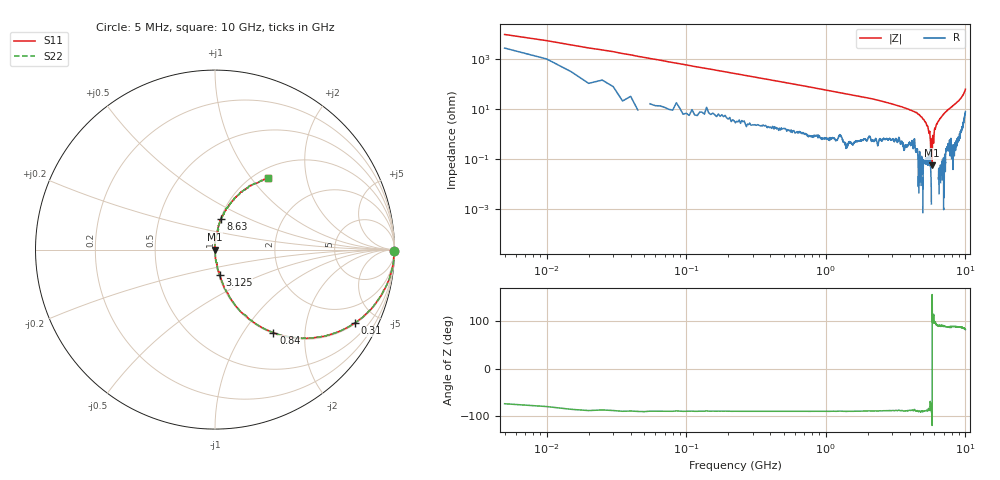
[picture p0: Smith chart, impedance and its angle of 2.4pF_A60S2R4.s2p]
! Amotech Co.,Ltd.
! http://www.amotech.co.kr/
! Part Number: A60S2R4
! These Parameters are Measured in Series Mode Connection
! Operation Temp=25[degC], DC Bias Voltage=0[V]
! Freq. Start=5[MHz] Stop=10[GHz], 2000[Steps]
! Date: Monday, July 13, 2020, 01:52:19
# GHZ S RI R 50.000000
!Freq.(Hz) S11(Real) S11(Imag) S21(Real) S21(Imag) S12(Real) S12(Imag) S22(Real) S22(Imag)
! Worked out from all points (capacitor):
!   2000 points, 5 MHz to 10 GHz, reference 50 ohm
!   read as one part in series: C = 2.74 pF near 55 MHz
!   lowest |Z| = 54.2 mohm at 5.785 GHz (marker M1)
!   series resonance near 5.784 GHz, so ESL is about 280 pH
!   S11 on the Smith chart (normalised r, x): 5 MHz: open; 310 MHz: 1.05, -3.78; 840 MHz: 1.02, -1.38; 3.125 GHz: 1.01, -0.29; 8.63 GHz: 1.01, +0.35; 10 GHz: 1.16, +1.22
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0.005  0.997 -0.00986  0.00304 0.00986  0.00304 0.00986  0.997 -0.00986
0.065  0.9863 -0.1091  0.0137 0.1091  0.0137 0.1091  0.9863 -0.1091
0.105  0.9668 -0.1742  0.0332 0.1742  0.0332 0.1742  0.9668 -0.1742
0.31  0.7781 -0.4094  0.2219 0.4094  0.2219 0.4094  0.7781 -0.4094
0.84  0.325 -0.4621  0.675 0.4621  0.675 0.4621  0.325 -0.4621
1.675  0.1039 -0.2975  0.8961 0.2975  0.8961 0.2975  0.1039 -0.2975
3.125  0.0262 -0.1419  0.9738 0.1419  0.9738 0.1419  0.0262 -0.1419
3.34  0.0236 -0.1266  0.9764 0.1266  0.9764 0.1266  0.0236 -0.1266
4.465  0.00768 -0.0724  0.9923 0.0724  0.9923 0.0724  0.00768 -0.0724
5.005  0.00214 -0.0382  0.9979 0.0382  0.9979 0.0382  0.00214 -0.0382
5.55  0.000747 -0.0128  0.9993 0.0128  0.9993 0.0128  0.000747 -0.0128
5.66  0.000245 -0.000822  0.9998 0.000822  0.9998 0.000822  0.000245 -0.000822
5.72  -5.15e-05 -0.00556  1 0.00556  1 0.00556  -5.15e-05 -0.00556
5.785  -0.000497 0.000219  1 -0.000219  1 -0.000219  -0.000497 0.000219
5.85  -0.000891 0.00841  1.001 -0.00841  1.001 -0.00841  -0.000891 0.00841
5.93  -0.0018 0.00438  1.002 -0.00438  1.002 -0.00438  -0.0018 0.00438
6.035  -0.00168 0.0167  1.002 -0.0167  1.002 -0.0167  -0.00168 0.0167
6.67  0.00153 0.0444  0.9985 -0.0444  0.9985 -0.0444  0.00153 0.0444
8.335  0.0238 0.1481  0.9762 -0.1481  0.9762 -0.1481  0.0238 0.1481
8.63  0.0332 0.17  0.9668 -0.17  0.9668 -0.17  0.0332 0.17
9.53  0.1119 0.2887  0.8881 -0.2887  0.8881 -0.2887  0.1119 0.2887
10  0.2963 0.3969  0.7037 -0.3969  0.7037 -0.3969  0.2963 0.3969
